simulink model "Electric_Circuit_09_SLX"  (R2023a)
settings: Solver=ode23s  StartTime=0.0  StopTime=10.0  MaxStep=0.001  RelTol=1e-3
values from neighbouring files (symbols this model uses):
  C_4 = 0.001*F    (= 0.001)    [Electric_Circuit_09_EQN.m]    (also in Electric_Circuit_09_SLX_m.m; Electric_Circuit_01_EQN.m; Electric_Circuit_01_SLX_m.m; Electric_Circuit_06_EQN.m)
  I_2_0 = 0*A    (= 0)    [Electric_Circuit_09_SLX_m.m]    (also in Electric_Circuit_02_SLX_m.m; Electric_Circuit_03_SLX_m.m; Electric_Circuit_06_SLX_m.m; Electric_Circuit_08_SLX_m.m)
  I_5_0 = 0*A    (= 0)    [Electric_Circuit_09_SLX_m.m]    (also in BIG_EC_Simscape_SLX_m.m; Electric_Circuit_01_SLX_m.m; Electric_Circuit_06_SLX_m.m; Electric_Circuit_10_SLX_m.m)
  I_7_0 = 0*A    (= 0)    [Electric_Circuit_09_SLX_m.m]    (also in Electric_Circuit_01_SLX_m.m; Inductive_Circuit_2_SLX_m.m)
  L_2 = 0.002*H    (= 0.002)    [Electric_Circuit_09_EQN.m]    (also in Electric_Circuit_09_SLX_m.m; Electric_Circuit_02_EQN.m; Electric_Circuit_02_SLX_m.m; Electric_Circuit_03_EQN.m)
  L_5 = 0.002*H    (= 0.002)    [Electric_Circuit_09_EQN.m]    (also in Electric_Circuit_09_SLX_m.m; BIG_EC_Simscape_EQN.m; BIG_EC_Simscape_SLX_m.m; Electric_Circuit_01_EQN.m)
  L_7 = 0.002*H    (= 0.002)    [Electric_Circuit_09_EQN.m]    (also in Electric_Circuit_09_SLX_m.m; Inductive_Circuit_2_EQN.m; Inductive_Circuit_2_SLX_m.m)
  R_3 = 100*Ohm    (= 100)    [Electric_Circuit_09_EQN.m]    (also in Electric_Circuit_09_SLX_m.m; Electric_Circuit_01_EQN.m; Electric_Circuit_01_SLX_m.m; Electric_Circuit_02_EQN.m)
  R_6 = 100*Ohm    (= 100)    [Electric_Circuit_09_EQN.m]    (also in Electric_Circuit_09_SLX_m.m; BIG_EC_Simscape_EQN.m; BIG_EC_Simscape_SLX_m.m; Electric_Circuit_02_EQN.m)
  Ts = Tfin/Nr_Ts_Points    (= 0.00014997)    [Electric_Circuit_09_SLX_m.m]    (also in BIG_EC_Simscape_SLX_m.m = 0.0003; Car_Dumper_SLX_m.m = 0.0022779; Electric_Circuit_01_SLX_m.m = 0.005; Electric_Circuit_02_SLX_m.m = 0.000480145)
  V_1_0 = 10*V    (= 10)    [Electric_Circuit_09_SLX_m.m]    (also in BIG_EC_Simscape_SLX_m.m; Electric_Circuit_02_SLX_m.m; Electric_Circuit_03_SLX_m.m; Electric_Circuit_04_SLX_m.m)
  V_4_0 = 0*V    (= 0)    [Electric_Circuit_09_SLX_m.m]    (also in Electric_Circuit_01_SLX_m.m; Electric_Circuit_06_SLX_m.m)
  V_8_0 = 0*V    (= 0)    [Electric_Circuit_09_SLX_m.m]    (also in BIG_EC_Simscape_SLX_m.m; Electric_Circuit_03_SLX_m.m; Electric_Circuit_04_SLX_m.m; Electric_Circuit_11_SLX_m.m)

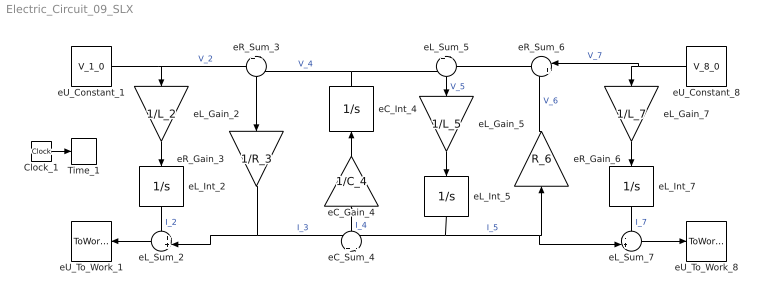
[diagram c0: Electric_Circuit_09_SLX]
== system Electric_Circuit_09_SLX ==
  Clock_1 : Clock
  Time_1 : ToWorkspace  VariableName=t  SaveFormat=Timeseries  SampleTime=Ts
  eC_Gain_4 : Gain  Gain=1/C_4  Multiplication=Matrix(K*u)
  eC_Int_4 : Integrator  InitialCondition=V_4_0
  eC_Sum_4 : Sum  Inputs=+|-
  eL_Gain_2 : Gain  Gain=1/L_2  Multiplication=Matrix(K*u)
  eL_Gain_5 : Gain  Gain=1/L_5  Multiplication=Matrix(K*u)
  eL_Gain_7 : Gain  Gain=1/L_7  Multiplication=Matrix(K*u)
  eL_Int_2 : Integrator  InitialCondition=I_2_0
  eL_Int_5 : Integrator  InitialCondition=I_5_0
  eL_Int_7 : Integrator  InitialCondition=I_7_0
  eL_Sum_2 : Sum  Inputs=++|
  eL_Sum_5 : Sum  Inputs=+|-
  eL_Sum_7 : Sum  Inputs=-+|
  eR_Gain_3 : Gain  Gain=1/R_3  Multiplication=Matrix(K*u)
  eR_Gain_6 : Gain  Gain=R_6  Multiplication=Matrix(K*u)
  eR_Sum_3 : Sum  Inputs=+|-
  eR_Sum_6 : Sum  Inputs=|++
  eU_Constant_1 : Constant  Value=V_1_0
  eU_Constant_8 : Constant  Value=V_8_0
  eU_To_Work_1 : ToWorkspace  VariableName=I_1_0  SaveFormat=Timeseries  SampleTime=Ts
  eU_To_Work_8 : ToWorkspace  VariableName=I_8_0  SaveFormat=Timeseries  SampleTime=Ts
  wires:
  eR_Gain_3/1 -> eL_Sum_2/2, eC_Sum_4/1  "I_3"
  eL_Sum_2/1 -> eU_To_Work_1/1
  eU_Constant_1/1 -> eL_Gain_2/1, eR_Sum_3/1  "V_2"
  eL_Gain_2/1 -> eL_Int_2/1
  eL_Int_2/1 -> eL_Sum_2/1  "I_2"
  eC_Int_4/1 -> eR_Sum_3/2, eL_Sum_5/1  "V_4"
  eR_Sum_3/1 -> eR_Gain_3/1
  eL_Int_5/1 -> eC_Sum_4/2, eR_Gain_6/1, eL_Sum_7/2  "I_5"
  eC_Sum_4/1 -> eC_Gain_4/1  "I_4"
  eC_Gain_4/1 -> eC_Int_4/1
  eR_Sum_6/1 -> eL_Sum_5/2
  eL_Sum_5/1 -> eL_Gain_5/1  "V_5"
  eL_Gain_5/1 -> eL_Int_5/1
  eU_Constant_8/1 -> eR_Sum_6/1, eL_Gain_7/1  "V_7"
  eR_Gain_6/1 -> eR_Sum_6/2  "V_6"
  eL_Sum_7/1 -> eU_To_Work_8/1
  eL_Gain_7/1 -> eL_Int_7/1
  eL_Int_7/1 -> eL_Sum_7/1  "I_7"
  Clock_1/1 -> Time_1/1
